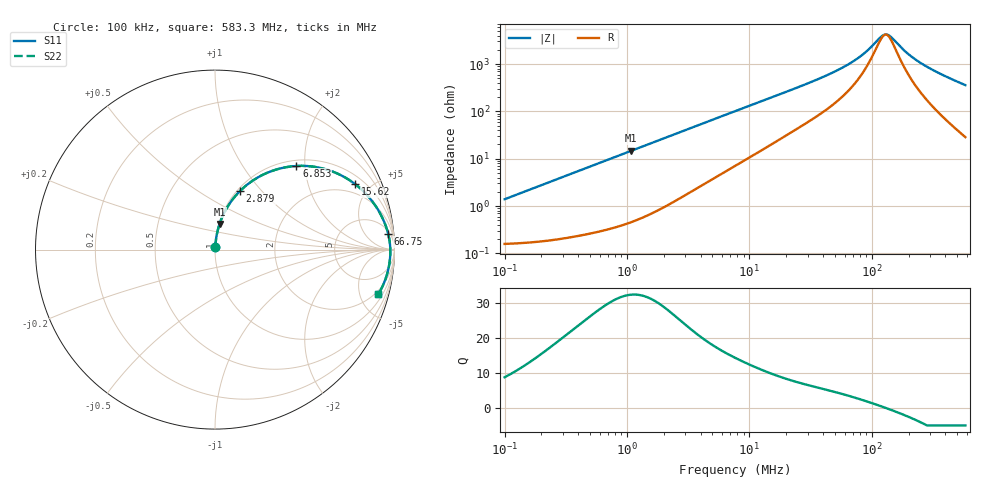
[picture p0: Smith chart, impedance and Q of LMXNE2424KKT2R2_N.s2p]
! LMXNE2424KKT2R2_N  S-PARAMETER MODEL  ( General Type )
! Model Generated by TAIYO YUDEN Corporation (https://www.yuden.co.jp/en/)
! Version 1.0
! TAIYO YUDEN Control No. 191023NI43SB-FBB
! Copyright(c) 2019 TAIYO YUDEN CO.,LTD. All Rights Reserved.
! Product Description (link to TY-COMPAS)
! https://ds.yuden.co.jp/TYCOMPAS/or/detail?pn=LMXNE2424KKT2R2MN&u=M
! Products Name : Inductors
! Characteristics :
!  Inductance : 2.2 uH , SRF(min) : 77 MHz , DC Resistance(max) : 0.18 Ohm
!  Rated Current : Saturation :1290 mA , Temp Rise : 970 mA (40 degC)
!  Case Size : 2.4 x 2.4 / 0.095 x 0.095 [mm/inch] , Thickness : 1 / 0.039 [mm/inch]
!  (Conditions: Temperature = 25 degC , DC Bias Current/Voltage = 0A / 0V)
! External Node Assignments :
!  1  o---GGG---o  2
! GND o---------o GND
! Frequency Range : 0.1MHz  -  583.332491MHz  [ 402 STEP ]
# MHz S RI R 50
! Freq[MHz].  S11 Real  S11 Imag  S21 Real  S21 Imag  S12 Real  S12 Imag  S22 Real  S22 Imag
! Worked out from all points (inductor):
!   401 points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, 100 kHz to 583.3 MHz, reference 50 ohm
!   read as one part in series: L = 2.2 uH near 104.4 kHz
!   highest Q = 32.3 at 1.085 MHz (marker M1), where L = 2.16 uH
!   self-resonance near 130.2 MHz
!   S11 on the Smith chart (normalised r, x): 100 kHz: 1.00, +0.03; 2.879 MHz: 1.03, +0.77; 6.853 MHz: 1.12, +1.81; 15.62 MHz: 1.42, +4.02; 66.75 MHz: 7, +20; 583.3 MHz: 1.57, -7.14
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0.1  0.00177 0.0138  0.9982 -0.0138  0.9982 -0.0138  0.00177 0.0138
0.427357  0.00578 0.058  0.9942 -0.058  0.9942 -0.058  0.00578 0.058
1.085493  0.0255 0.1428  0.9745 -0.1428  0.9745 -0.1428  0.0255 0.1428
1.826341  0.0643 0.229  0.9357 -0.229  0.9357 -0.229  0.0643 0.229
2.879337  0.1403 0.3273  0.8597 -0.3273  0.8597 -0.3273  0.1403 0.3273
4.346839  0.2625 0.4149  0.7375 -0.4149  0.7375 -0.4149  0.2625 0.4149
6.853054  0.4532 0.4659  0.5468 -0.4659  0.5468 -0.4659  0.4532 0.4659
7.637621  0.5026 0.4662  0.4974 -0.4662  0.4974 -0.4662  0.5026 0.4662
10.57255  0.6446 0.4387  0.3554 -0.4387  0.3554 -0.4387  0.6446 0.4387
15.61875  0.7805 0.365  0.2195 -0.365  0.2195 -0.365  0.7805 0.365
22.09443  0.8617 0.2871  0.1383 -0.2871  0.1383 -0.2871  0.8617 0.2871
32.63992  0.9179 0.2054  0.0821 -0.2054  0.0821 -0.2054  0.9179 0.2054
49.27539  0.9514 0.1324  0.0486 -0.1324  0.0486 -0.1324  0.9514 0.1324
66.74783  0.9652 0.0866  0.0348 -0.0866  0.0348 -0.0866  0.9652 0.0866
88.4768  0.9727 0.0485  0.0273 -0.0485  0.0273 -0.0485  0.9727 0.0485
122.4761  0.9765 0.00754  0.0235 -0.00754  0.0235 -0.00754  0.9765 0.00754
130.706  0.9768 -0.000527  0.0232 0.000527  0.0232 0.000527  0.9768 -0.000527
139.489  0.9769 -0.00861  0.0231 0.00861  0.0231 0.00861  0.9769 -0.00861
193.0909  0.9751 -0.0503  0.0249 0.0503  0.0249 0.0503  0.9751 -0.0503
250.4606  0.9702 -0.087  0.0298 0.087  0.0298 0.087  0.9702 -0.087
370.0033  0.954 -0.152  0.046 0.152  0.046 0.152  0.954 -0.152
583.3325  0.9106 -0.2481  0.0894 0.2481  0.0894 0.2481  0.9106 -0.2481
